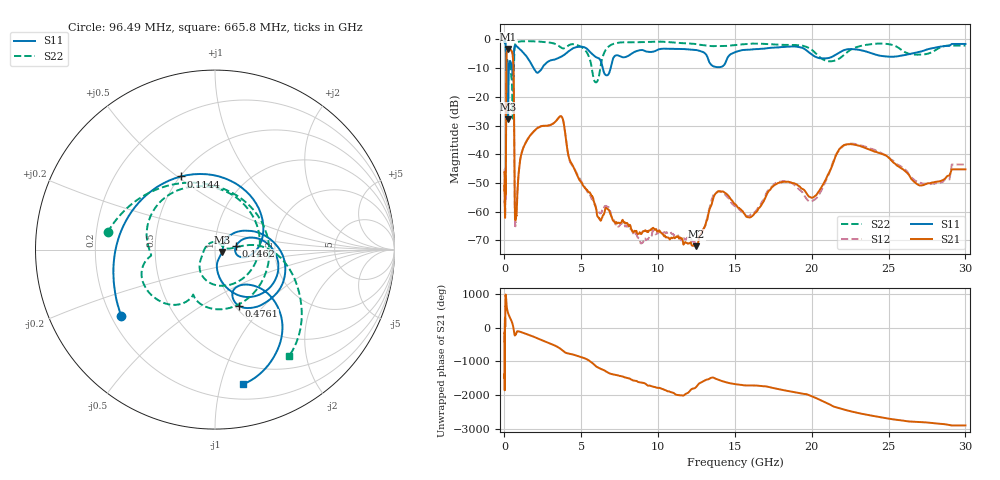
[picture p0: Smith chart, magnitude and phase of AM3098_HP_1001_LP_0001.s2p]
! Date/Time: Thu, Feb 28, 2019 8:40 AM
! Network Analyzer: Agilent Technologies E8364B Rev: A.07.50.67
! Sweep from 0.010 to 30.000 GHz, 1601 Points, Sweep Type: LOG
! Power Supply: 5.023 V, 0.002 A
# Hz S DB R 50
!freq MagS11 AngS11 MagS21 AngS21 MagS12 AngS12 MagS22 AngS22
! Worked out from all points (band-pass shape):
!   1601 points, 10 MHz to 30 GHz, reference 50 ohm
!   highest |S21| = -3.30 dB at 237.5 MHz (marker M1); lowest = -72.0 dB at 12.5 GHz (marker M2)
!   |S21| within 3 dB of the highest: 129.4 MHz to 550.9 MHz (421.5 MHz wide, 124 % of centre)
!   lowest |S11| = -27.8 dB at 237.5 MHz (marker M3), VSWR 1.09, Z = 54 - j1.35 ohm
!   |S11| at or under -10 dB: 198.7 MHz to 290.5 MHz (91.87 MHz wide, 37.6 % of centre); 1.897 GHz to 2.441 GHz (544.2 MHz wide, 25.1 % of centre); 6.392 GHz to 6.911 GHz (518.7 MHz wide, 7.8 % of centre)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
!   |S22| runs from -27.6 to -0.5 dB; largest |S21 - S12| = 0.009
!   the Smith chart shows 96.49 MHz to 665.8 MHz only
!   S11 on the Smith chart (normalised r, x): 96.49 MHz: 0.24, -0.30; 114.4 MHz: 0.50, +0.51; 146.2 MHz: 1.27, +0.06; 476.1 MHz: 1.04, -0.74; 665.8 MHz: 0.32, -1.18
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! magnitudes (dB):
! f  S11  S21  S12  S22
! 10 MHz  -0.4  -46.2  -45.2  -0.5
! 38.04 MHz  -0.5  -61.2  -59.1  -0.8
! 96.49 MHz  -3.9  -43.4  -43.0  -4.3
! 114.4 MHz  -6.9  -16.7  -16.6  -10.4
! 144.7 MHz  -18.8  -4.4  -4.4  -10.6
! 146.2 MHz  -18.4  -4.4  -4.3  -10.4
! 190.6 MHz  -9.0  -3.8  -3.8  -7.2
! 237.5 MHz  -27.8  -3.3  -3.3  -8.9
! 299 MHz  -9.2  -3.5  -3.5  -7.9
! 476.1 MHz  -9.3  -4.1  -4.1  -14.0
! 550.5 MHz  -11.9  -6.3  -6.2  -27.3
! 605.4 MHz  -5.6  -15.6  -15.6  -11.6
! 665.8 MHz  -2.3  -54.0  -55.0  -2.8
! 717.7 MHz  -2.1  -62.4  -63.8  -1.5
! 2.084 GHz  -11.5  -31.1  -31.1  -0.7
! 3.704 GHz  -6.0  -26.8  -26.8  -2.9
! 5.959 GHz  -6.2  -58.9  -58.8  -15.0
! 7.926 GHz  -6.1  -64.1  -65.3  -1.0
! 12.5 GHz  -3.7  -72.0  -70.2  -1.6
! 20.1 GHz  -5.6  -55.0  -56.1  -4.1
! 22.56 GHz  -3.4  -36.5  -36.3  -3.5
! 30 GHz  -1.6  -45.3  -43.6  -2.1
